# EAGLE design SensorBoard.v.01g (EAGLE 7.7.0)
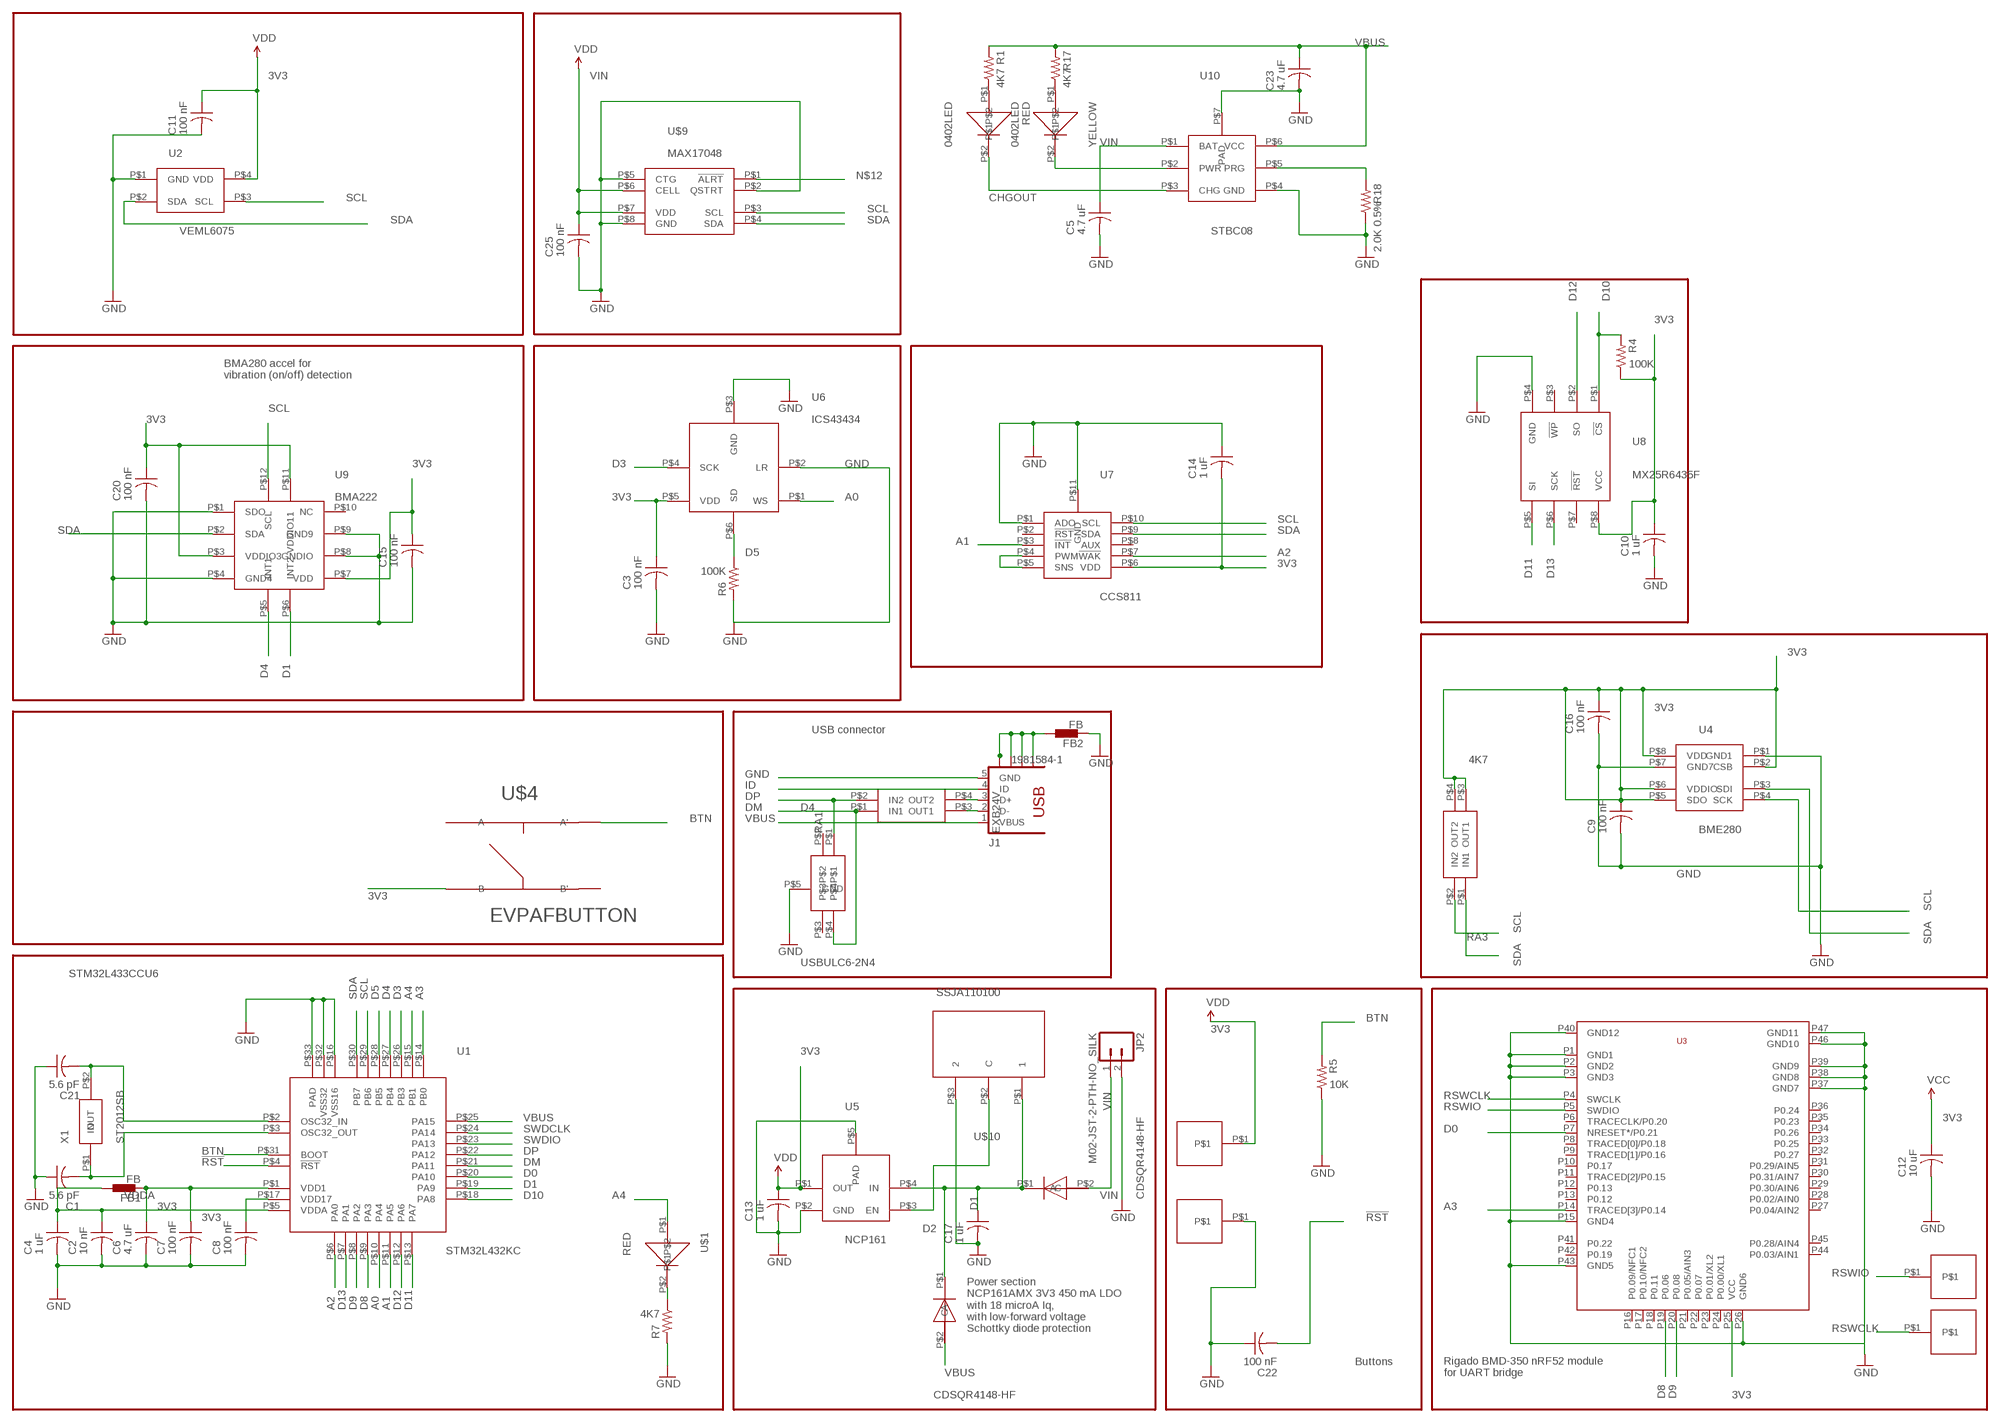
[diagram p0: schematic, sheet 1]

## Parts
C1  5.6 pF  C-US  [C0402_B]
C2  10 nF  C-US  [C0402_B]
C3  100 nF  C-US  [C0402_B]
C4  1 uF  C-US  [C0402_B]
C5  4.7 uF  C-US  [C0402_B]
C6  4.7 uF  C-US  [C0402_B]
C7  100 nF  C-US  [C0402_B]
C8  100 nF  C-US  [C0402_B]
C9  100 nF  C-US  [C0402_B]
C10  1 uF  C-US  [C0402_B]
C11  100 nF  C-US  [C0402_B]
C12  10 uF  C-US  [C0402_B]
C13  1 uF  C-US  [C0402_B]
C14  1 uF  C-US  [C0402_B]
C15  100 nF  C-US  [C0402_B]
C16  100 nF  C-US  [C0402_B]
C17  1 uF  C-US  [C0402_B]
C20  100 nF  C-US  [C0402_B]
C21  5.6 pF  C-US  [C0402_B]
C22  100 nF  C-US  [C0402_B]
C23  4.7 uF  C-US  [C0402_B]
C25  100 nF  C-US  [C0402_B]
D1  CDSQR4148-HF  [CDSQR4148-HF]
D2  CDSQR4148-HF  [CDSQR4148-HF]
D4  USBULC6-2N4  [USBULC6-2N4]
FB1  FB  BLM15H  [0402]
FB2  FB  BLM15H  [0402]
J1  1981584-1  [1981584-1]
JP2  M02-JST-2-PTH-NO_SILK  [JST-2-PTH-NS]
R1  4K7  R-US_  [R0402_B]
R4  100K  R-US_  [R0402_B]
R5  10K  R-US_  [R0402_B]
R6  100K  R-US_  [R0402_B]
R7  4K7  R-US_  [R0402_B]
R17  4K7  R-US_  [R0402_B]
R18  2.0K 0.5%  R-US_  [R0402_B]
RA1  EXB24V  [EXB24V]
RA3  4K7  EXB24V  [EXB24V]
RED  0402LED  [0402LED]
U1  STM32L432KC  [STM32L432KC]
U2  VEML6075  [A3OP]
U3  BMD-350  [BMD-350]
U4  BME280  [BME280]
U5  NCP161  [NCP161]
U6  ICS43434  [ICS43434]
U7  CCS811  [CCS811]
U8  MX25R6435F  [MX25R6435F]
U9  BMA222  [BMA222]
U10  STBC08  [STBC08]
U$1  RED  0402LED  [0402LED]
U$2  HN01  [HN01]
U$3  HN01  [HN01]
U$4  EVPAFBUTTON  [EVPAF-BUTTON-SPDT]
U$7  HN01  [HN01]
U$8  HN01  [HN01]
U$9  MAX17048  [MAX17048]
U$10  SSJA110100  [SSAJ110100]
X1  ST2012SB  [ST2012SB]
YELLOW  0402LED  [0402LED]

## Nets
3V3: C3.1 C6.1 C7.1 C8.1 C9.1 C10.1 C11.1 C12.1 C13.1 C14.2 C15.1 C16.1 C20.1 FB1.1 R4.1 RA3.P$3(OUT1) RA3.P$4(OUT2) U1.P$1(VDD1) U1.P$17(VDD17) U2.P$4(VDD) U3.P25(VCC) U4.P$2(CSB) U4.P$5(SDO) U4.P$6(VDDIO) U4.P$8(VDD) U5.P$1(OUT) U6.P$5(VDD) U7.P$6(VDD) U8.P$8(VCC) U9.P$3(VDDIO3) U9.P$7(VDD) U9.P$11(VDDIO11) U$2.P$1 U$4.P$3(B) ; supply symbol labelled VDD, VCC
!RST: C22.2 U1.P$4(!RST)
A0: U1.P$10(PA4) U6.P$1(WS)
A1: U1.P$11(PA5) U7.P$3(!INT)
A2: U1.P$6(PA0) U7.P$7(!WAK)
A3: U1.P$14(PB0) U3.P14(TRACED[3]/P0.14)
A4: U1.P$15(PB1) U$1.P$1
BTN: R5.2 U1.P$31(BOOT) U$4.P$2(A')
CHGOUT: RED.P$2 U10.P$3(CHG)
D0: U1.P$20(PA10) U3.P7(NRESET*/P0.21)
D1: U1.P$19(PA9) U9.P$6(INT2)
D3: U1.P$26(PB3) U6.P$4(SCK)
D4: U1.P$27(PB4) U9.P$5(INT1)
D5: R6.1 U1.P$28(PB5) U6.P$6(SD)
D8: U1.P$9(PA3) U3.P19(P0.06)
D9: U1.P$8(PA2) U3.P20(P0.08)
D10: R4.2 U1.P$18(PA8) U8.P$1(!CS)
D11: U1.P$13(PA7) U8.P$5(SI)
D12: U1.P$12(PA6) U8.P$2(SO)
D13: U1.P$7(PA1) U8.P$6(SCK)
DM: D4.P$4 RA1.P$1(IN1) U1.P$21(PA11)
DP: D4.P$1 RA1.P$2(IN2) U1.P$22(PA12)
GND: C1.1 C2.2 C3.2 C4.2 C5.2 C6.2 C7.2 C8.2 C9.2 C10.2 C11.2 C12.2 C13.2 C14.1 C15.2 C16.2 C17.2 C20.2 C21.1 C22.1 C23.2 C25.2 D4.P$5(GND) FB2.1 J1.5(GND) JP2.2 R5.1 R6.2 R7.2 R18.1 U1.P$16(VSS16) U1.P$32(VSS32) U1.P$33(PAD) U2.P$1(GND) U3.P1(GND1) U3.P2(GND2) U3.P3(GND3) U3.P15(GND4) U3.P26(GND6) U3.P37(GND7) U3.P38(GND8) U3.P39(GND9) U3.P40(GND12) U3.P43(GND5) U3.P46(GND10) U3.P47(GND11) U4.P$1(GND1) U4.P$7(GND7) U5.P$2(GND) U5.P$5(PAD) U6.P$2(LR) U6.P$3(GND) U7.P$1(ADO) U7.P$11(GND) U8.P$4(GND) U9.P$1(SDO) U9.P$4(GND4) U9.P$8(GNDIO) U9.P$9(GND9) U10.P$4(GND) U10.P$7(PAD) U$3.P$1 U$9.P$2(QSTRT) U$9.P$5(CTG) U$9.P$8(GND) U$10.P$3
ID: J1.4(ID)
N$1: R7.1 U$1.P$2
N$2: U5.P$3(EN) U$10.P$2(C)
N$3: C21.2 U1.P$2(OSC32_IN) X1.P$2(OUT)
N$4: C1.2 U1.P$3(OSC32_OUT) X1.P$1(IN)
N$10: U7.P$4(PWM) U7.P$5(SNS)
N$12: U$9.P$1(!ALRT)
N$13: U10.P$2(PWR) YELLOW.P$2
N$15: R1.1 RED.P$1
N$17: R17.1 YELLOW.P$1
N$27: R18.2 U10.P$5(PRG)
N$31: J1.3(D+) RA1.P$4(OUT2)
N$33: J1.2(D-) RA1.P$3(OUT1)
N$60: C17.1 D1.P$1(C) D2.P$1(C) U5.P$4(IN) U$10.P$1
RSWCLK: U3.P4(SWCLK) U$8.P$1
RSWIO: U3.P5(SWDIO) U$7.P$1
SCL: RA3.P$2(IN2) U1.P$29(PB6) U2.P$3(SCL) U4.P$4(SCK) U7.P$10(SCL) U9.P$12(SCL) U$9.P$3(SCL)
SDA: RA3.P$1(IN1) U1.P$30(PB7) U2.P$2(SDA) U4.P$3(SDI) U7.P$9(SDA) U9.P$2(SDA) U$9.P$4(SDA)
SWDCLK: U1.P$24(PA14)
SWDIO: U1.P$23(PA13)
USB_SHIELD: FB2.2 J1.S1 J1.S2 J1.S3 J1.S4
VBUS: C23.1 D2.P$2(A) J1.1(VBUS) R1.2 R17.2 U1.P$25(PA15) U10.P$6(VCC)
VDDA: C2.1 C4.1 FB1.2 U1.P$5(VDDA)
VIN: C5.1 C25.1 D1.P$2(A) JP2.1 U10.P$1(BAT) U$9.P$6(CELL) U$9.P$7(VDD) ; supply symbol labelled VDD
Unconnected: D4.P$2 D4.P$3 U3.P6(TRACECLK/P0.20) U3.P8(TRACED[0]/P0.18) U3.P9(TRACED[1]/P0.16) U3.P10(P0.17) U3.P11(TRACED[2]/P0.15) U3.P12(P0.13) U3.P13(P0.12) U3.P16(P0.09/NFC1) U3.P17(P0.10/NFC2) U3.P18(P0.11) U3.P21(P0.05/AIN3) U3.P22(P0.07) U3.P23(P0.01/XL2) U3.P24(P0.00/XL1) U3.P27(P0.04/AIN2) U3.P28(P0.02/AIN0) U3.P29(P0.30/AIN6) U3.P30(P0.31/AIN7) U3.P31(P0.29/AIN5) U3.P32(P0.27) U3.P33(P0.25) U3.P34(P0.26) U3.P35(P0.23) U3.P36(P0.24) U3.P41(P0.22) U3.P42(P0.19) U3.P44(P0.03/AIN1) U3.P45(P0.28/AIN4) U7.P$2(!RST) U7.P$8(AUX) U8.P$3(!WP) U8.P$7(!RST) U9.P$10(NC) U$4.P$1(A) U$4.P$4(B')

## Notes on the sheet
- BMA280 accel for
  vibration (on/off) detection
- USB connector
- STM32L433CCU6
- Power section
  NCP161AMX 3V3 450 mA LDO
  with 18 microA Iq, 
  with low-forward voltage 
  Schottky diode protection
- Buttons
- Rigado BMD-350 nRF52 module
  for UART bridge

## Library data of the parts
C1-C17 C20-C23 C25 = Spark:C-US: Capacitor
D1 D2 = Kris:CDSQR4148-HF: ComChip's CDSQR4148-HF high speed 150 mA Io diode
D4 = Kris:USBULC6-2N4: ST TVS diode ESD Protection USBULC6-2N4
FB1 FB2 = STM32L433SARA.AssetTracker.v01:BLM15H: EMIFIL (R) Chip Ferrite Bead for GHz Noise
J1 = con-usb:1981584-1: Receptacle, micro-USB, type A/B Tyco Electronics; MF: Hirose; MPN: ZX62-AB-5PA(11)
JP2 = SparkFun-Connectors:M02: Standard 2-pin 0.1" header. Use with
R1 R4-R7 R17 R18 = Spark:R-US_: 0402 Resistor
RA1 RA3 = Kris:EXB24V: Panasonic EXB24 22 Ohm series resistor pair
RED U$1 YELLOW = Kris:0402LED: 0402led
U1 = STM32L432KC:STM32L432KC: STM32L432KC UFQFPN32 - 32-pin, 5x5 mm, 0.5 mm pitch ultra thin fine pitch quad flat package http://www.st.com/content/ccc/resource/technical/document/datasheet/24/01/9f/59/f0/83/47/fc/DM00257205.pdf/files/DM00257205.pdf/jcr:content/translations/en.DM00257205.pdf
U2 = Kris:VEML6075: A3OP package for VEML6040 and VEML6075 Vishay light sensors
U3 = BMD-350-Eagle:BMD-350
U4 = Kris:BME280: BME280 Bosch pressure, humidity, temperature sensor
U5 = Kris:NCP161: NCP161 3V3 LDO voltage regulator
U6 = Invensense:ICS43434: ICS43434 I2S Digital Microphone
U7 = Kris:CCS811: CCS811 Air Quality Sensor http://ams.com/eng/Products/Environmental-Sensors/Gas-Sensors/CCS811
U8 = Kris:MX25R6435F: MX25R6435F 64 MBit SPI NOR Flash from Macronix
U9 = Kris:BMA222: Bosch BMA222 3-axis accelerometer
U10 = Kris:STBC08: STBC08 800 mA standalone LiPo battery charger
U$2 U$3 U$7 U$8 = PWSONN6:HN01
U$4 = SparkFun-Electromechanical:EVPAFBUTTON: EVPAF Momentary switch by panasonic
U$9 = Kris:MAX17048: MAX17048 LiPo Battery Fuel Gauge
U$10 = Kris:SSJA110100: ALPS SSJA110100 SPDT slide switch with lugs
X1 = Kris:ST2012SB: Kyocera 2.0 x 1.2 mm 32.768 20kHz ppm 4 pf crystal

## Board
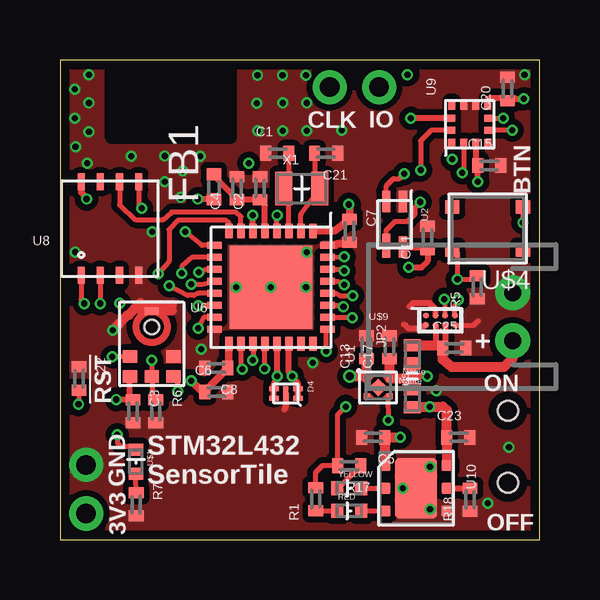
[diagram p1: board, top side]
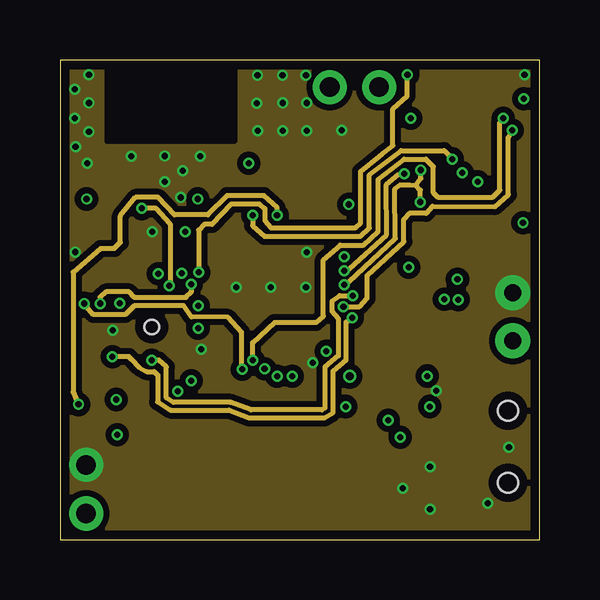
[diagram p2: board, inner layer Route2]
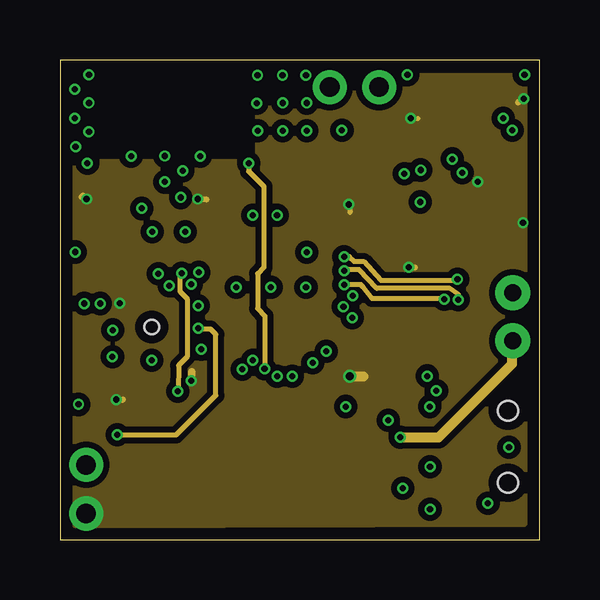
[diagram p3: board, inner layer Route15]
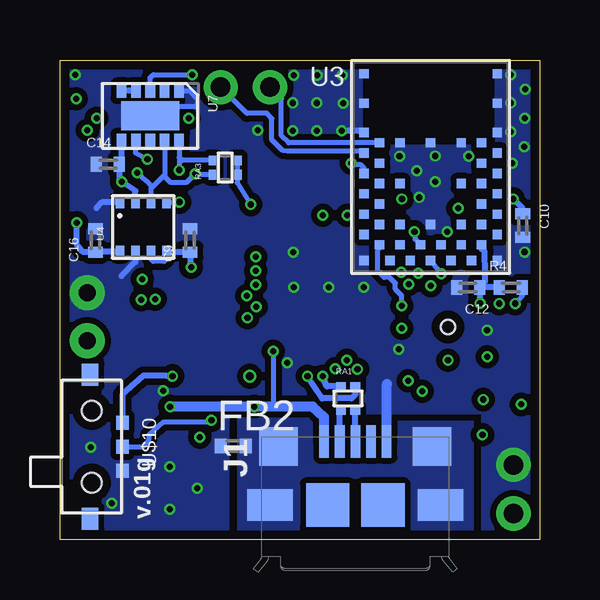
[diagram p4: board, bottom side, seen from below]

Size 19.99 x 19.99 mm. Coordinates in mm from the lower left corner, seen from the top.
Outline: 0,0 19.99,0 19.99,19.99 0,19.99 0,0
Copper layers (1*2*15*16): Top 0.035559375mm / dielectric 0.17018125mm / Route2 0.01778125mm / dielectric 47mil / Route15 0.01778125mm / dielectric 0.17018125mm / Bottom 0.035559375mm
Design rules "OSHPark-4layer *": minimum track width 5mil, minimum drill 10mil, track to track 5mil, track to pad 5mil, pad to pad 5mil, via to via 5mil, smd to smd 5mil, copper to edge 15mil, drill to drill 6mil, minimum pad ring 4mil, minimum via ring 4mil, stop-mask expansion 4mil, vias tented up to drill 20mil, thermal gap 10mil

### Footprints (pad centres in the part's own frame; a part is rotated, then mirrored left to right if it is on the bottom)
C0402_B = smd 0.457 x 0.61: 1 -0.483,0; 2 0.483,0
CDSQR4148-HF = smd 0.7 x 0.5: P$1 0,0.375; P$2 0,-0.375
USBULC6-2N4 = smd 0.2 x 0.4: P$1 0.2,0.5; P$2 -0.2,0.5; P$3 -0.2,-0.5; P$4 0.2,-0.5 | smd 0.6 x 0.2: P$5 0,0
0402 = smd 0.5 x 0.61: 1 -0.5,0; 2 0.55,0
1981584-1 = smd 0.4 x 1.35: 1 -1.3,4.1; 2 -0.65,4.1; 3 0,4.1; 4 0.65,4.1; 5 1.3,4.1 | smd 1.8 x 1.8: M1 -1.15,1.45; M2 1.15,1.45 | smd 1.9 x 1.3: S1 -3.55,1.45; S2 3.55,1.45 | smd 1.6 x 1.6: S3 -3.2,3.885; S4 3.2,3.885
JST-2-PTH-NS = drill 0.7 pad 1.448: 1 -1,0; 2 1,0
R0402_B = smd 0.457 x 0.61: 1 -0.483,0; 2 0.483,0
EXB24V = smd 0.4 x 0.36: P$1 -0.3,0.5; P$2 0.3,0.5; P$3 -0.3,-0.5; P$4 0.3,-0.5
0402LED = smd 0.5 x 0.6: P$1 -0.5,0; P$2 0.5,0
STM32L432KC = smd 0.6 x 0.3: P$1 -2.35,1.75; P$2 -2.35,1.25; P$3 -2.35,0.75; P$4 -2.35,0.25; P$5 -2.35,-0.25; P$6 -2.35,-0.75; P$7 -2.35,-1.25; P$8 -2.35,-1.75; P$17 2.35,-1.75; P$18 2.35,-1.25; P$19 2.35,-0.75; P$20 2.35,-0.25; P$21 2.35,0.25; P$22 2.35,0.75; P$23 2.35,1.25; P$24 2.35,1.75 | smd 0.3 x 0.6: P$9 -1.75,-2.35; P$10 -1.25,-2.35; P$11 -0.75,-2.35; P$12 -0.25,-2.35; P$13 0.25,-2.35; P$14 0.75,-2.35; P$15 1.25,-2.35; P$16 1.75,-2.35; P$25 1.75,2.35; P$26 1.25,2.35; P$27 0.75,2.35; P$28 0.25,2.35; P$29 -0.25,2.35; P$30 -0.75,2.35; P$31 -1.25,2.35; P$32 -1.75,2.35 | smd 3.45 x 3.45: P$33 0,0
A3OP = smd 0.9 x 0.35: P$1 -0.95,0.35; P$2 -0.95,-0.35; P$4 0.95,0.35 | smd 1 x 0.35: P$3 0.9,-0.35
BMD-350 = smd 0.39 x 0.39: P1 0.425,8.2; P2 0.425,6.975; P3 0.425,5.75; P4 1.075,5.325; P5 0.425,4.9; P6 1.075,4.475; P7 0.425,4.05; P8 1.075,3.625; P9 0.425,3.2; P10 1.075,2.775; P11 0.425,2.35; P12 1.075,1.925; P13 0.425,1.5; P14 1.075,1.075; P15 0.425,0.425; P16 1.5,0.425; P17 1.925,1.075; P18 2.35,0.425; P19 2.775,1.075; P20 3.2,0.425; P21 3.625,1.075; P22 4.05,0.425; P23 4.475,1.075; P24 4.9,0.425; P25 5.325,1.075; P26 5.975,0.425; P27 5.975,1.5; P28 5.325,1.925; P29 5.975,2.35; P30 5.325,2.775; P31 5.975,3.2; P32 5.325,3.625; P33 5.975,4.05; P34 5.325,4.475; P35 5.975,4.9; P36 5.325,5.325; P37 5.975,5.75; P38 5.975,6.975; P39 5.975,8.2; P40 1.925,5.325; P41 1.925,3.625; P42 1.925,1.925; P43 3.2,1.925; P44 4.475,1.925; P45 4.475,3.625; P46 4.475,5.325; P47 3.2,5.325
BME280 = smd 0.5 x 0.35: P$1 1.025,0.975; P$2 1.025,0.325; P$3 1.025,-0.325; P$4 1.025,-0.975; P$5 -1.025,-0.975; P$6 -1.025,-0.325; P$7 -1.025,0.325; P$8 -1.025,0.975
NCP161 = smd 0.24 x 0.24: P$1 -0.37,-0.48; P$2 0.37,-0.48; P$3 0.37,0.48; P$4 -0.37,0.48 | smd 0.52 x 0.52 rotated 45: P$5 0,0
ICS43434 = smd 0.6 x 0.522: P$1 0.9,-1.364; P$2 0.9,-0.532; P$4 -0.9,-0.532; P$5 -0.9,-1.364; P$6 0,-1.364 | smd 0.6 x 0.3: P$3 0,1.368 | hole 0.6: 0,0.7
CCS811 = smd 0.6 x 0.4: P$1 -1.05,1.2; P$2 -1.05,0.6; P$3 -1.05,0; P$4 -1.05,-0.6; P$5 -1.05,-1.2; P$6 1.05,-1.2; P$7 1.05,-0.6; P$8 1.05,0; P$9 1.05,0.6; P$10 1.05,1.2 | smd 1.2 x 2.4: P$11 0,0
MX25R6435F = smd 0.3 x 0.7: P$1 1.2,1.95; P$2 0.4,1.95; P$3 -0.4,1.95; P$4 -1.2,1.95; P$5 -1.2,-1.95; P$6 -0.4,-1.95; P$7 0.4,-1.95; P$8 1.2,-1.95
BMA222 = smd 0.41 x 0.28: P$1 -0.815,0.75; P$2 -0.815,0.25; P$3 -0.815,-0.25; P$4 -0.815,-0.75; P$7 0.815,-0.75; P$8 0.815,-0.25; P$9 0.815,0.25; P$10 0.815,0.75 | smd 0.28 x 0.41: P$5 -0.25,-0.815; P$6 0.25,-0.815; P$11 0.25,0.815; P$12 -0.25,0.815
STBC08 = smd 0.45 x 0.5: P$1 -0.95,-1.3; P$2 0,-1.3; P$3 0.95,-1.3; P$4 0.95,1.3; P$5 0,1.3; P$6 -0.95,1.3 | smd 2.5 x 1.75: P$7 0,0
HN01 = drill 0.813 pad 1.422: P$1 0,0
EVPAF-BUTTON-SPDT = smd 0.6 x 0.55: P$1 -1.475,0.9; P$2 1.475,0.9; P$3 -1.475,-0.9; P$4 1.475,-0.9
MAX17048 = smd 0.25 x 0.25: P$1 -0.6,0.2; P$2 -0.2,0.2; P$3 0.2,0.2; P$4 0.6,0.2; P$5 -0.6,-0.2; P$6 -0.2,-0.2; P$7 0.2,-0.2; P$8 0.6,-0.2
SSAJ110100 = smd 0.6 x 0.51: P$1 -1,1.28; P$2 0,1.285; P$3 1,1.285 | smd 0.9 x 0.7: P$4 3,-0.07; P$5 -3,-0.07 | hole 0.83: -1.5,0; 1.5,0
ST2012SB = smd 0.7 x 1.4: P$1 -0.75,0; P$2 0.75,0

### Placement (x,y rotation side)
C1  9.06,16.1 0 top
C2  8.33,14.64 90 top
C3  3.04,5.36 270 top
C4  7.38,14.64 90 top
C5  13.06,4.27 180 top
C6  6.52,6.16 0 top
C7  12.06,12.88 270 top
C8  6.52,7.16 180 top
C9  14.57,12.47 90 bottom
C10  0.71,13.09 270 bottom
C11  15.32,12.57 90 top
C12  2.98,10.52 180 bottom
C13  12.78,8.03 90 top
C14  18,15.65 0 bottom
C15  17.88,15.6 0 top
C16  18.52,12.47 90 bottom
C17  13.73,8.03 90 top
C20  18.64,18.78 90 top
C21  11.09,16.1 180 top
C22  0.79,6.72 270 top
C23  16.6,4.27 0 top
C25  16.42,7.99 0 top
D1  14.68,7.73 180 top
D2  14.68,5.91 0 top
D4  9.41,6.1 270 top
FB1  6.41,14.68 90 top
FB2  12.8,3.91 0 bottom
J1  7.68,0 0 bottom
JP2  18.86,9.3 90 top
R1  10.66,1.69 90 top
R4  1.21,10.52 0 bottom
R5  17.39,10.52 90 top
R6  3.99,5.36 270 top
R7  3.17,1.47 270 top
R17  12.05,3.09 180 top
R18  17.08,1.66 90 top
RA1  7.99,5.89 0 bottom
RA3  13.11,15.51 90 bottom
RED  12.05,1.21 0 top
U1  8.79,10.52 270 top
U2  13.94,13.14 270 top
U3  7.75,11.21 0 bottom
U4  16.52,13.03 90 bottom
U5  13.26,6.35 270 top
U6  3.82,8.17 0 top
U7  16.23,17.67 270 bottom
U8  2.08,12.97 180 top
U9  17.07,17.31 90 top
U10  14.83,2.15 270 top
U$1  3.16,3.25 270 top
U$2  1.09,1.09 90 top
U$3  1.09,3.12 0 top
U$4  17.82,12.97 180 top
U$7  13.3,18.86 0 top
U$8  11.24,18.86 0 top
U$9  15.85,9.14 0 top
U$10  18.67,3.87 270 bottom
X1  10.07,14.63 0 top
YELLOW  12.05,2.15 0 top

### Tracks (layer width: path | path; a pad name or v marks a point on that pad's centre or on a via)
3V3  (via drill 0.25, 0.33)
  Top 0.203: 1.4,0.79 U$2.P$1 | U$4.P$3 19.29,13.96 | 2.88,6.76 U6.P$5
  Top 0.254: U9.P$11 v14.62,17.56 | 19.29,13.96 19.29,13.23 v19.29,13.21 | U2.P$4 15.21,12.19 C11.1 15.32,11.61 15.06,11.35 v14.53,11.35 | U8.P$8 0.88,14.47 v1.1,14.2 | v2.35,5.84 C3.1 2.88,5.99 2.88,6.76 | U9.P$7 17.82,18.29 17.82,18.37 17.91,18.41 18.49,18.41 C20.1 18.97,18.38 v19.32,18.38 | 17.42,15.65 C15.1 | U9.P$3 17.32,15.78 C15.1 | v17.41,14.92 17.41,15.68 C15.1 | FB1.1 5.89,14.19 v5.74,14.2
  Top 0.305: U1.P$17 7.04,7.25 C8.1 C6.1 5.92,6.16 v5.47,6.63 | U1.P$1 11.46,12.87 C7.1 12.06,13.89 v12.04,13.97
  Top 0.406: C13.1 U5.P$1 12.69,6.81 v12.08,6.81
  Route15 0.203: v12.04,13.97 12.09,13.64 | v14.62,17.56 14.91,17.55 | v1.1,14.2 0.89,14.28
  Route15 0.254: v19.29,13.21 19.27,13.17 19.28,13.13 | v14.53,11.35 14.8,11.35 | 0.89,14.28 0.95,14.34 | v2.35,5.84 2.63,5.84 | v19.32,18.38 19.13,18.26 19.07,18.21 | v5.74,14.2 6.11,14.19
  Route15 0.305: v5.47,6.63 5.49,7
  Route15 0.406: v12.08,6.81 12.65,6.81
  Bottom 0.203: U4.P$6 | v12.04,13.97 12.61,14.87 RA3.P$3 RA3.P$4
  Bottom 0.254: U3.P25 2.42,12.12 2.31,12.01 2.3,11.09 2.3,10.72 C12.1 | 17.44,14.87 v17.41,14.92 | v19.29,13.21 19.29,12.31 19.05,12.01 18.53,12.01 C16.1 18.5,12.01 U4.P$8 | U4.P$2 16.85,14.54 v17.41,14.92 | U4.P$6 16.19,11.71 16.1,11.62 15.66,11.62 15.55,11.74 U4.P$5 14.58,12.01 C9.1 14.57,11.39 v14.53,11.35 | v17.41,14.92 17.51,14.86 C14.2 17.43,15.73 U7.P$6 | C10.1 0.71,13.8 v1.1,14.2 | R4.1 C12.1 | C12.1 2.5,9.87 v2.49,9.86
  pour Route15 (isolate 0.254, no thermals): 0.64,19.35 19.35,19.35 19.35,0.64 0.64,0.57
!RST  (via drill 0.25)
  Top 0.203: U1.P$4 v9.04,13.52 v9.04,13.53 | C22.2 0.79,5.66 v0.77,5.64
  Route2 0.203: v9.04,13.53 9.04,13.84 8.5,14.34 6.96,14.34 6.16,13.54 4.78,13.54 4.1,14.26 3.14,14.26 2.52,13.5 2.52,12.39 2.26,12.14 1.69,12.14 0.55,11.15 0.55,6.15 v0.77,5.64
A0  (via drill 0.25)
  Top 0.203: U1.P$10 5.5,11.77 5.08,11.39 v5.07,11.1 | v4.9,6.18 4.9,6.56 U6.P$1
  Route15 0.203: v5.07,11.1 5,10.94 5,10.34 5.3,10.05 5.3,7.63 4.94,7.26 4.93,6.21 v4.9,6.18
A1  (via drill 0.25)
  Top 0.203: U1.P$11 6.12,11.27 v5.78,11.14
  Route2 0.203: v14.48,19.38 14.46,19.23 14.46,18.49 13.87,17.96 13.87,16.42 13.44,16.09 13.3,15.98 12.52,15.35 12.52,13.21 12.29,12.99 8.79,12.99 8.53,13.3 8.53,13.79 8.31,13.99 7.15,13.99 6.34,13.14 6.01,13.14 5.78,12.9 v5.78,11.14
  Bottom 0.203: U7.P$3 16.23,19.25 16.1,19.38 v14.48,19.38
A2  (via drill 0.25)
  Top 0.254: U1.P$6 8.04,13.46 v8.03,13.53
  Route2 0.203: v16.34,15.86 16,16.22 14.21,16.22 12.89,15.2 12.89,12.99 12.51,12.64 8.52,12.64 8.03,13.09 v8.03,13.53
  Bottom 0.203: U7.P$7 16.84,16.11 v16.34,15.86
A3  (via drill 0.25)
  Top 0.203: U1.P$14 6.15,9.75 v5.75,9.75
  Bottom 0.203: U3.P14 6.67,12.18 6.77,12.03 6.77,11.24 6.49,10.94 6.26,10.94 6.02,10.69 6.02,10.44 5.75,10.17 v5.75,9.75
A4  (via drill 0.25)
  Top 0.203: U1.P$15 6,9.27 v5.75,8.81 | v2.39,4.37 2.39,4.04 2.52,3.9 3.03,3.9 U$1.P$1
  Route15 0.203: v2.39,4.37 4.84,4.37 6.49,6.02 6.49,8.56 6.27,8.78 5.79,8.78 v5.75,8.81
BTN  (via drill 0.25)
  Top 0.203: U1.P$31 11.66,11.76 v11.84,11.8 | U$4.P$2 16.34,12.16 16.56,11.94 v16.56,10.86 17.21,10.86 R5.2
  Route15 0.203: v11.84,11.8 12.05,11.8 12.26,11.6 12.65,11.6 13.37,10.81 16.47,10.81 v16.56,10.86
CHGOUT
  Top 0.203: RED.P$2 U10.P$3
D0  (via drill 0.25)
  Top 0.203: v8.52,7.12 8.53,7.33 U1.P$20
  Route15 0.203: v7.86,15.68 7.86,15.35 8.5,14.72 8.5,11.35 8.23,11.09 8.23,9.63 8.53,9.32 8.53,7.14 v8.52,7.12
  Bottom 0.203: U3.P7 7.32,15.49 7.46,15.62 7.8,15.62 v7.86,15.68
D1  (via drill 0.25)
  Top 0.203: U1.P$19 8.05,7.67 v8.04,7.48 | U9.P$6 v18.47,17.56
  Route2 0.203: v8.04,7.48 8.03,8.22 8.94,9.05 10.67,9.05 10.97,9.32 10.97,11.66 11.67,12.28 12.64,12.28 13.26,12.85 13.26,15.01 14.34,15.86 15.24,15.86 15.56,15.54 15.56,14.45 15.75,14.28 18.02,14.28 18.33,14.57 18.31,17.36 v18.47,17.56
D3  (via drill 0.25)
  Top 0.203: v12.18,9.25 11.16,9.25 U1.P$26 | U6.P$4 2.56,7.63 v2.18,7.62
  Route2 0.203: v12.18,9.25 11.93,9.07 11.93,7.49 11.38,7.04 11.38,5.3 11.02,5.08 7.87,5.08 7.05,5.4 4.6,5.4 4.06,5.74 4.08,6.86 3.92,7.01 3.61,7.01 3.29,7.19 3,7.51 2.87,7.63 v2.18,7.62
D4  (via drill 0.25)
  Top 0.203: v18.85,17.07 18.68,17.06 U9.P$5 | U1.P$27 11.75,9.77 v11.81,9.71
  Route2 0.203: v18.85,17.07 18.67,16.75 18.68,14.38 18.12,13.88 15.53,13.89 15.51,13.89 15.25,13.6 14.55,13.6 14.33,13.36 14.33,12.42 12.8,11.01 12.8,10.06 12.48,9.72 11.89,9.72 v11.81,9.71
D5  (via drill 0.25)
  Top 0.203: U1.P$28 11.5,10.27 11.65,10.17 v12.21,10.17 | v3.82,7.48 U6.P$6 3.83,6.79 3.83,5.99 R6.1
  Route2 0.203: v3.82,7.48 4.12,7.48 4.43,7.2 4.43,5.91 4.73,5.73 7.11,5.73 7.96,5.41 10.92,5.41 11.04,5.5 11.04,7.19 11.6,7.66 11.6,9.21 11.33,9.51 11.33,9.93 11.65,10.17 v12.21,10.17
D8  (via drill 0.25)
  Top 0.203: U1.P$9 5.92,12.27 v5.22,12.84
  Bottom 0.203: v5.22,12.84 5.19,12.51 U3.P19
D9  (via drill 0.25)
  Top 0.203: U1.P$8 7.04,13.21 6.91,13.31 4.92,13.31 4.55,12.93 4.55,11.6 v4.1,11.09
  Bottom 0.203: U3.P20 4.55,11.6 v4.1,11.09
D10  (via drill 0.25)
  Top 0.203: U1.P$18 7.54,7.19 v7.59,7.1 | U8.P$1 0.88,10.01 v1.02,9.84
  Route2 0.203: v7.59,7.1 7.57,7.09 7.57,8.65 7.01,9.27 5.47,9.28 5.16,9.75 3.1,9.74 2.71,9.38 1.39,9.38 v1.02,9.84
  Bottom 0.203: R4.2 0.72,10.17 v1.02,9.84
D11  (via drill 0.25)
  Top 0.203: U1.P$13 5.74,10.27 5.58,10.19 5.31,10.19 v4.55,10.58 | U8.P$5 3.28,13.94 v3.4,13.8
  Route2 0.203: v3.4,13.8 4,13.8 4.58,13.16 4.58,10.62 v4.55,10.58
D12  (via drill 0.25)
  Top 0.203: v5.46,10.64 5.93,10.64 U1.P$12 | U8.P$2 v1.68,9.84
  Route2 0.203: v5.46,10.64 5.46,10.31 5.25,10.1 3.1,10.1 3.1,10.11 2.88,10.32 1.92,10.32 1.68,10.11 v1.68,9.84
D13
  Top 0.203: U1.P$7 7.54,13.47 7.32,13.65 4.65,13.65 4.29,13.34 3.14,13.34 2.48,13.95 U8.P$6
DM  (via drill 0.25)
  Top 0.254: D4.P$4 8.91,6.39 v9.04,6.82 | v9.04,6.82 9.05,6.89 9.05,7.03 | 9.05,7.03 9.05,8.16 U1.P$21 | v9.04,6.82 9.06,6.91 9.05,7.03
  Bottom 0.254: RA1.P$1 8.87,6.39 v9.04,6.82
DP  (via drill 0.25)
  Top 0.254: U1.P$22 9.54,6.99 9.91,6.5 D4.P$1 9.91,6.51 v9.68,6.81
  Bottom 0.254: RA1.P$2 7.69,6.04 7.84,5.89 9.06,5.89 v9.68,6.81
GND  (via drill 0.25)
  Top 0.203: U$9.P$2 15.65,9.66 | U$9.P$8 17.24,8.94 17.44,9.12
  Top 0.254: D4.P$5 9.41,5.59 9.36,5.42 | 15.48,9.78 15.65,9.61 U$9.P$2 15.65,9.6 15.39,9.86 14.71,9.86 14.57,9.72 | U$9.P$5 15.21,8.94 15.06,8.8 14.52,8.8 14.34,8.98 | U6.P$3 4.66,9.53 4.66,9.54 4.66,9.7 3.42,9.7 3.33,9.61 3.33,9.49 3.34,9.47 4.69,9.47 4.75,9.54 4.75,9.84 4.74,9.86 3.35,9.86 | 2.87,9.37 2.83,9.37
  Top 0.305: U1.P$32 11.49,12.27 11.56,12.33 12,12.33 C7.2
  Top 0.406: 3.35,9.86 2.87,9.37 | 2.83,9.37 v2.2,8.74
  Bottom 0.203: U7.P$1 14.59,18.72 14.28,18.34 14.28,18.12 14.36,18.03 15.8,18.03 15.89,18.01 U7.P$11
  Bottom 0.254: U4.P$1 18.24,14.05 18.48,13.82 | U4.P$7 16.85,11.57 17.44,10.99 | U3.P3 7.41,16.96 7.49,17.04 v8.24,17.04
  Bottom 0.406: J1.5 6.37,6.49
  other vias: 8.79,10.52 7.34,10.52 2.96,15.98 5.84,15.98 8.19,18.19 8.23,19.35 9.27,19.35 9.28,18.2 9.28,17.04 0.61,18.77 1.21,18.2 1.21,16.99 10.25,19.35 10.29,18.2 10.29,17.04 11.75,17.06 10.27,11.98 10.25,10.52 14.27,2.15 17.83,1.52 15.68,6.21 19.35,19.38 10.53,7.38 5.88,7.94 0.62,17.56 18.71,3.86 1.21,19.38 4.36,15.99 5.03,14.26 3.85,12.84 0.65,16.38 1.14,15.68 0.64,11.99 5.12,15.38 4.36,14.91 15.42,3.04 15.42,1.27
  pour Top (isolate 0.254, no thermals): 0,19.99 19.99,19.99 19.99,0 0,0
  pour Route2 (isolate 0.254, no thermals): 0,19.99 19.99,19.99 19.99,0 0,0
  pour Bottom (isolate 0.254, no thermals): 2.35,0 0,0 0,19.99 19.99,19.99 19.99,0 13.02,0 13.02,5.33 2.35,5.33
  pour Top (no thermals): 2.98,9.72 4.61,9.72 2.97,9.7
N$1
  Top 0.203: R7.1 3.16,2.6 U$1.P$2
N$2  (via drill 0.25)
  Top 0.203: U5.P$3 13.66,5.98 v13.68,4.98
  Bottom 0.203: U$10.P$2 16.55,3.87 16.29,4.14 16.29,4.36 15.66,4.92 13.78,4.92 13.69,4.93 v13.68,4.98
N$3
  Top 0.203: U1.P$2 10.04,13.56 X1.P$2 10.6,14.85 C21.2
N$4
  Top 0.203: U1.P$3 9.54,14.17 X1.P$1 9.54,14.85 C1.2
N$5
  cutout Route2: 1.97,19.95 7.28,19.96 7.28,16.59 1.97,16.59
N$6
  cutout Route15: 1.88,19.96 8.01,19.96 8.01,15.95 1.33,15.95 1.33,19.94
N$7
  cutout Bottom: 15.24,14.35 17.83,14.35 17.83,11.73 15.23,11.73 15.23,14.35
N$8
  cutout Bottom: 14.87,18.34 15.33,18.34 15.33,18.12 14.87,18.12
N$10
  Bottom 0.254: U7.P$4 U7.P$5
N$13
  Top 0.203: YELLOW.P$2 U10.P$2
N$15
  Top 0.203: R1.1 RED.P$1
N$17
  Top 0.203: YELLOW.P$1 11.6,2.15 R17.1
N$27
  Top 0.254: U10.P$5 R18.2
N$31
  Bottom 0.254: J1.3 7.68,5.27 RA1.P$4
N$33
  Bottom 0.254: J1.2 8.33,5.23 RA1.P$3
N$60  (via drill 0.25)
  Top 0.254: v15.3,6.82 14.91,6.82 14.6,6.81
  Top 0.406: D2.P$1 14.59,6.57 | 14.59,6.57 14.6,6.81 D1.P$1 | 14.59,6.57 14.59,6.72 U5.P$4 13.74,7.52 C17.1
  Bottom 0.254: v15.3,6.82 15.58,6.83 16.52,6.83 17.39,6.06 17.39,4.91 U$10.P$1
RSWCLK
  Bottom 0.203: U3.P4 10.47,16.54 10.77,16.84 10.77,18.39 U$8.P$1
RSWIO
  Bottom 0.203: U$7.P$1 12.21,17.77 11.35,17.77 11.16,17.55 11.16,16.66 10.7,16.22 10.51,16.19 7.54,16.19 7.44,16.11 U3.P5
SCL  (via drill 0.25)
  Top 0.203: U1.P$29 11.57,10.77 v11.84,10.63 | U$9.P$3 16.05,9.97 v16.02,10.02 | U2.P$3 13.6,12.9 13.97,13.27 14.49,13.27 14.8,13.58 14.8,13.86 v15.01,14.07 | U9.P$12 15.47,17.06 U7.P$10 15.03,15.41 v15.02,15.4
  Route2 0.203: v11.84,10.63 12.03,10.74 13.97,12.56 13.96,14.62 14.17,14.78 14.57,14.78 14.83,14.78 | 14.83,14.78 15.03,15.05 v15.02,15.4 | v15.01,14.07 15.01,14.57 14.83,14.78
  Route15 0.203: v16.02,10.02 15.93,10.05 13.01,10.05 12.64,10.52 12.54,10.63 v11.84,10.63
  Bottom 0.203: U7.P$10 15.02,15.93 | 15.02,15.93 15.02,15.56 v15.02,15.4 | U4.P$4 15.1,14.05 v15.01,14.07 | RA3.P$2 14.9,15.81 15.02,15.93
SDA  (via drill 0.25)
  Top 0.203: U1.P$30 11.76,11.27 v11.84,11.21 | U$9.P$4 16.45,9.76 v16.6,10.01 | U9.P$2 16.82,15.31 v16.76,15.29 16.71,15.24 | U2.P$2 13.6,14.74 13.89,15.04 14.14,15.04 v14.35,15.25
  Route2 0.203: v11.84,11.21 12.05,11.29 13.61,12.71 13.6,14.8 14.08,15.2 14.34,15.2 14.34,15.24 v14.35,15.25
  Route15 0.203: v16.6,10.01 16.6,10.22 16.24,10.48 13.21,10.48 12.46,11.25 11.87,11.25 v11.84,11.21
  Bottom 0.203: 16.14,14.7 16.4,14.96 v16.76,15.29 | U7.P$9 15.63,15.21 | 15.63,15.21 16.14,14.7 | U4.P$3 16.2,14.64 16.14,14.7 | v14.35,15.25 14.38,15.32 | 15.63,15.21 15.63,15.12 15.4,14.9 14.71,14.9 v14.35,15.25 | RA3.P$1 14.3,15.21 v14.35,15.25
USB_SHIELD
  pour Bottom (isolate 0.254, rank 3, no thermals): 2.86,0 2.86,5.21 12.51,5.21 12.51,0
VBUS  (via drill 0.25)
  Top 0.203: v11.1,7.85 11.1,8.73 U1.P$25 | R1.2 10.65,2.81 10.95,3.1 11.56,3.1 R17.2 11.57,5.22 v11.9,5.55
  Top 0.406: 14.54,5.51 D2.P$2 14.83,5.54 v15.4,5.55 15.96,5.55 16.12,5.4 C23.1 16.13,4.25 U10.P$6
  Bottom 0.203: v11.1,7.85 11.1,5.86 11.09,5.55
  Bottom 0.406: J1.1 8.98,5.11 9.45,5.55 11.09,5.55 v11.9,5.55 v15.4,5.55
VDDA
  Top 0.254: U1.P$5 8.54,13.93 C2.1 C4.1 6.43,15.18 FB1.2
VIN  (via drill 0.25)
  Top 0.254: U$9.P$7 16.05,8.09 C25.1 16.05,8.1 15.97,8.1 | U$9.P$6 15.65,8.13 15.64,8.1
  Top 0.406: JP2.1 18.86,7.56 18.49,7.19 16.32,7.19 15.94,7.51 C25.1 | D1.P$2 15.64,8.1 15.97,8.1 | U10.P$1 C5.1 v14.17,4.27
  Route15 0.406: v14.17,4.27 15.77,4.27 18.83,7.33 18.83,8.27 JP2.1

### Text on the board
tPlace: CLK | IO | BTN | !RST | + | ON | GND | STM32L432 / SensorTile | OFF | 3V3
bPlace: v.01g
